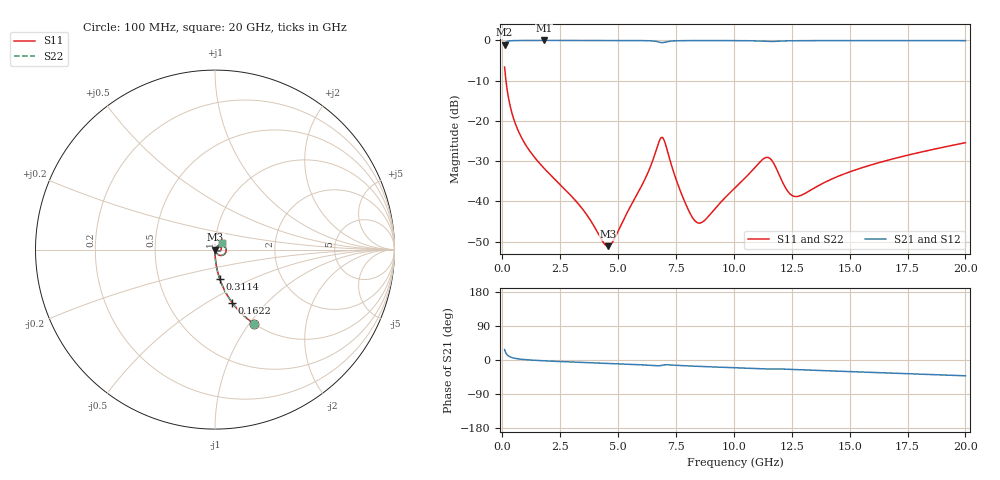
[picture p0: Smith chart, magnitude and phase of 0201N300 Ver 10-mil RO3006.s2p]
# GHz S MA R 50
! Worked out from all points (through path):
!   1601 points, 100 MHz to 20 GHz, reference 50 ohm
!   highest |S21| = -0.02 dB at 1.804 GHz (marker M1); lowest = -1.1 dB at 100 MHz (marker M2)
!   group delay of S21, straight-line fit = 6.15 ps
!   lowest |S11| = -51.1 dB at 4.565 GHz (marker M3), VSWR 1.01, Z = 50.3 - j0.0653 ohm
!   |S11| at or under -10 dB: 158.6 MHz to end of sweep
!   |S22| runs from -51.1 to -6.6 dB; largest |S21 - S12| = 0
!   S11 on the Smith chart (normalised r, x): 100 MHz: 1.00, -1.06; 162.2 MHz: 1.00, -0.65; 311.4 MHz: 1.00, -0.34; 20 GHz: 1.08, +0.08
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0.1  0.4673 -62.3  0.8834 27.7  0.8834 27.7  0.4673 -62.3
0.1621875  0.3097 -72.1  0.9501 17.7  0.9501 17.7  0.3097 -72.1
0.3114375  0.1668 -80.7  0.9852 9.0  0.9852 9.0  0.1668 -80.7
0.5353125  0.09729 -84.9  0.9943 4.5  0.9943 4.5  0.09729 -84.9
0.8338125  0.0617 -87.1  0.997 1.9  0.997 1.9  0.0617 -87.1
1.803937  0.02579 -88.6  0.998 -2.1  0.998 -2.1  0.02579 -88.6
3.420812  0.008339 -80.8  0.9976 -6.3  0.9976 -6.3  0.008339 -80.8
4.565062  0.00278 -13.5  0.9971 -9.0  0.9971 -9.0  0.00278 -13.5
4.813813  0.003322 18.0  0.9969 -9.6  0.9969 -9.6  0.003322 18.0
6.107312  0.01756 55.0  0.9931 -13.0  0.9931 -13.0  0.01756 55.0
6.741625  0.05263 23.5  0.9583 -15.2  0.9583 -15.2  0.05263 23.5
6.977938  0.05849 -25.6  0.9426 -13.1  0.9426 -13.1  0.05849 -25.6
7.786375  0.01148 -61.9  0.9919 -14.9  0.9919 -14.9  0.01148 -61.9
8.40825  0.005474 -19.5  0.9943 -16.6  0.9943 -16.6  0.005474 -19.5
8.744063  0.00584 10.9  0.9946 -17.4  0.9946 -17.4  0.00584 10.9
10.05  0.01473 44.8  0.9935 -20.6  0.9935 -20.6  0.01473 44.8
11.43056  0.03528 9.6  0.97 -23.6  0.97 -23.6  0.03528 9.6
11.67931  0.03108 -10.6  0.9694 -23.4  0.9694 -23.4  0.03108 -10.6
12.48775  0.01198 -3.1  0.9885 -24.8  0.9885 -24.8  0.01198 -3.1
13.37081  0.0141 33.5  0.9926 -26.9  0.9926 -26.9  0.0141 33.5
16.69162  0.03272 45.9  0.9935 -34.3  0.9935 -34.3  0.03272 45.9
20  0.05356 42.0  0.9922 -41.7  0.9922 -41.7  0.05356 42.0
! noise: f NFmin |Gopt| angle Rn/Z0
0.1  0.0005502  0.9224  0.2979  0.001569
2.301  0.004027  0.7748  4.61  0.003648
4.515  0.006984  0.7494  8.964  0.00558
6.729  0.03241  0.9123  13.32  0.08029
8.943  0.01334  0.7432  17.65  0.01018
11.14  0.02884  0.8443  21.92  0.03792
13.36  0.01905  0.7361  26.15  0.01371
15.57  0.01841  0.6921  30.29  0.01088
17.79  0.0197  0.6773  34.36  0.0108
20  0.02131  0.6694  38.37  0.01111
